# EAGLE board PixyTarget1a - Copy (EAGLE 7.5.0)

No outline drawn. Coordinates in mm, seen from the top.
Copper layers (1*16): Top 0.035mm / dielectric 1.5mm / Bottom 0.035mm
Design rules "default": minimum track width 10mil, minimum drill 0.6mm, track to track 8mil, track to pad 8mil, pad to pad 8mil, via to via 8mil, smd to smd 8mil, copper to edge 40mil, drill to drill 8mil, minimum pad ring 10mil, minimum via ring 8mil, stop-mask expansion 4mil, vias tented up to drill 0mil, thermal gap 10mil
Net classes: 0 default: width 0.406 mm; 1 ground: width 0.61 mm

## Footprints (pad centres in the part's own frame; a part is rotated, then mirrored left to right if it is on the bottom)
LED5MM = drill 0.813 octagon: A -1.27,0; K 1.27,0
R1206 = smd 1.6 x 1.803: 1 -1.422,0; 2 1.422,0
TSOP18XX = drill 0.813 long: GND -0.001,-0.027; OUT -2.501,-0.027; VCC 2.499,-0.027
6-PLCC = smd 3.5 x 1.5: P$1 -2.77,2.41; P$2 -2.77,0.29; P$3 -2.77,-1.78; P$4 3.03,-1.78; P$5 3.03,0.29; P$6 3.03,2.41
SOT-23-5 = smd 1 x 0.55: 1 -1.35,0.95; 2 -1.35,0; 3 -1.35,-0.95; 4 1.35,-0.95; 5 1.35,0.95
TEENSY_3.0-3.2&LC_DIL = drill 0.965: 0 -7.62,13.97; 1 -7.62,11.43; 2 -7.62,8.89; 3 -7.62,6.35; 3.3V 7.62,11.43; 4 -7.62,3.81; 5 -7.62,1.27; 6 -7.62,-1.27; 7 -7.62,-3.81; 8 -7.62,-6.35; 9 -7.62,-8.89; 10 -7.62,-11.43; 11 -7.62,-13.97; 12 -7.62,-16.51; 13 7.62,-16.51; 14/A0 7.62,-13.97; 15/A1 7.62,-11.43; 16/A2 7.62,-8.89; 17/A3 7.62,-6.35; 18/A4 7.62,-3.81; 19/A5 7.62,-1.27; 20/A6 7.62,1.27; 21/A7 7.62,3.81; 22/A8 7.62,6.35; 23/A9 7.62,8.89; AGND 7.62,13.97; GND -7.62,16.51; VIN 7.62,16.51

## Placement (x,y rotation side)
IR-TX  940NM  [LED5MM]  -8.89,-85.09 0 top
R1  120  [R1206]  -10.16,-91.44 0 top
R2  150  [R1206]  30.48,-72.39 0 top
R3  90  [R1206]  -3.81,-78.74 0 top
R4  150  [R1206]  -10.16,-78.74 0 top
R5  90  [R1206]  1.27,-78.74 0 top
R6  90  [R1206]  6.35,-78.74 0 top
R7  90  [R1206]  11.43,-78.74 0 top
R8  150  [R1206]  -10.16,-119.38 0 top
R9  90  [R1206]  -10.16,-125.73 0 top
R10  90  [R1206]  -3.81,-119.38 0 top
R11  150  [R1206]  -10.16,-142.24 0 top
R12  90  [R1206]  -3.81,-142.24 0 top
R13  90  [R1206]  -10.16,-148.59 0 top
U$1  MIDDLE  [TSOP18XX]  -7.62,-100.33 0 top
U$2  LED_RIGHT  [6-PLCC]  -7.62,-111.76 0 top
U$3  LED_RIGHT  [6-PLCC]  -7.62,-134.62 0 top
U$4  MIDDLE  [TSOP18XX]  27.94,-17.78 90 top
U$6  LED_RIGHT  [6-PLCC]  1.27,-54.61 0 top
U$7  LED_LEFT  [6-PLCC]  11.43,-54.61 0 top
U$8  QS5K2TR  [SOT-23-5]  21.59,-78.74 0 top
U$9  QS5K2TR  [SOT-23-5]  26.67,-78.74 0 top
U$10  QS5K2TR  [SOT-23-5]  16.51,-78.74 0 top
U$11  TEENSY_3.1-3.2_DIL  [TEENSY_3.0-3.2&LC_DIL]  -2.54,-31.75 0 top

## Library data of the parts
IR-TX = led
R1-R13 = resistor
U$1-U$4 U$6-U$10 = _Loper
U$11 = Teensy_3_and_LC_Series_Boards_v1.4

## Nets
+3V3: U$1.VCC U$4.VCC U$11.3.3V
+5V: R2.2 R3.2 R4.2 R5.2 R6.2 R7.2 R8.2 R9.2 R10.2 R11.2 R12.2 R13.2 U$11.VIN
BLU-L: U$8.3 U$11.17/A3
BLU-R: U$9.3 U$11.20/A6
GND [ground]: IR-TX.K U$1.GND U$4.GND U$8.2 U$9.2 U$10.2 U$11.AGND U$11.GND
GRN-L: U$10.1 U$11.16/A2
GRN-R: U$10.3 U$11.19/A5
IR-RX-1: U$1.OUT U$4.OUT U$11.4
IR-RX-2: U$11.6
IR-TX: R1.2 U$11.5
N$1: R8.1 U$2.P$1
N$2: R9.1 U$2.P$3
N$3: R2.1 U$7.P$1
N$4: R3.1 U$7.P$3
N$5: R6.1 U$7.P$2
N$6: U$7.P$5 U$10.5
N$7: R10.1 U$2.P$2
N$8: U$2.P$6 U$3.P$6 U$6.P$6 U$9.5
N$10: IR-TX.A R1.1
N$11: U$2.P$5 U$3.P$5 U$6.P$5 U$10.4
N$12: R11.1 U$3.P$1
N$13: R12.1 U$3.P$3
N$14: R13.1 U$3.P$2
N$19: U$7.P$4 U$8.4
N$20: U$7.P$6 U$8.5
N$25: R4.1 U$6.P$1
N$26: R5.1 U$6.P$3
N$28: R7.1 U$6.P$2
N$30: U$2.P$4 U$3.P$4 U$6.P$4 U$9.4
RED-L: U$8.1 U$11.15/A1
RED-R: U$9.1 U$11.18/A4

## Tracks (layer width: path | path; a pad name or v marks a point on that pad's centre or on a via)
+3V3  (2 unrouted)
+5V  (12 unrouted)
BLU-L  (1 unrouted)
BLU-R  (1 unrouted)
GND  (7 unrouted)
GRN-L  (1 unrouted)
GRN-R  (1 unrouted)
IR-RX-1  (2 unrouted)
IR-TX  (1 unrouted)
N$1  (1 unrouted)
N$2  (1 unrouted)
N$3  (1 unrouted)
N$4  (1 unrouted)
N$5  (1 unrouted)
N$6  (1 unrouted)
N$7  (1 unrouted)
N$8  (3 unrouted)
N$10  (1 unrouted)
N$11  (3 unrouted)
N$12  (1 unrouted)
N$13  (1 unrouted)
N$14  (1 unrouted)
N$19  (1 unrouted)
N$20  (1 unrouted)
N$25  (1 unrouted)
N$26  (1 unrouted)
N$28  (1 unrouted)
N$30  (3 unrouted)
RED-L  (1 unrouted)
RED-R  (1 unrouted)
